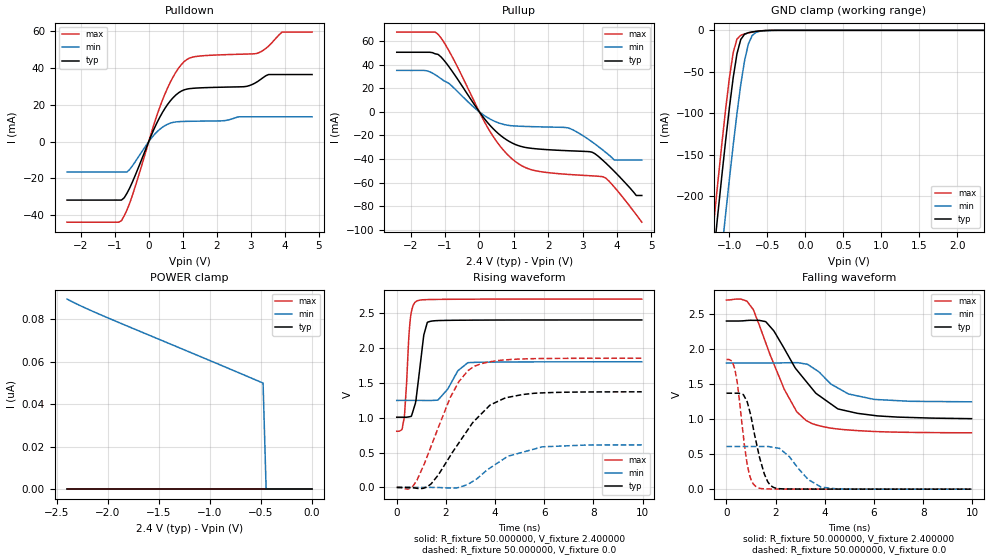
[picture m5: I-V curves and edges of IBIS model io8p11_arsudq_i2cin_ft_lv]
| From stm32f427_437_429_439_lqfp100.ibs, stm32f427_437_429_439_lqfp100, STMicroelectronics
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|   Model io8p11_arsudq_i2cin_ft_lv
[Model]  io8p11_arsudq_i2cin_ft_lv
Model_type I/O
Polarity   Non-Inverting
Enable   Active-Low
Vinl =   0.720000V
Vinh =   1.680000V
Vmeas =  1.200000V
Cref =   30.000000pF
Rref =   100.000000M
Vref =   0.0V
C_comp   2.230300pF   2.174000pF   2.332300pF
[Temperature Range]   25.000000   0.125000k   -40.000000
[Pullup Reference]   2.400000V   1.800000V   2.700000V
[Pulldown Reference]   0.0V   0.0V   0.0V
[POWER Clamp Reference]   2.400000V   1.800000V   2.700000V
[GND Clamp Reference]   0.0V   0.0V   0.0V
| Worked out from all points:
|   slope of the pulldown table from 0 to 0.36 V, typ, clamps not added: 25 ohm
|   slope of the pullup table from 0 to 0.36 V, typ, clamps not added: 27.7 ohm
|   GND clamp passes 1 mA (typ) near -0.62 V on its own axis
|   rising waveform, R_fixture 50.000000, V_fixture 2.400000: 20-80 % time 284ps typ, 604ps min, 184ps max; typ from 1.01 V to 2.4 V
|   rising waveform, R_fixture 50.000000, V_fixture 0.0: 20-80 % time 1.7ns typ, 1.69ns min, 1.31ns max; typ from 0 V to 1.37 V
|   falling waveform, R_fixture 50.000000, V_fixture 2.400000: 20-80 % time 1.81ns typ, 1.28ns min, 1.38ns max; typ from 2.4 V to 1.01 V
|   falling waveform, R_fixture 50.000000, V_fixture 0.0: 20-80 % time 535ps typ, 924ps min, 384ps max; typ from 1.37 V to 0 V
[Pulldown]
|Voltage   I(typ)   I(min)   I(max)
-2.4V     -31.73mA   -16.51mA   -43.74mA
-800mV    -31.73mA   -16.51mA   -42.87mA
-480mV    -21.98mA   -13.17mA   -29.21mA
80mV      3.63mA     1.966mA    5.014mA
480mV     18.16mA    8.738mA    26.02mA
800mV     25.38mA    10.72mA    37.77mA
1.12V     28.53mA    11.02mA    44.6mA
2.8V      29.84mA    13.49mA    47.53mA
3.2V      32.65mA    13.49mA    48.05mA
3.52V     36.43mA    13.49mA    51.84mA
3.92V     36.43mA    13.49mA    59.49mA
4.8V      36.43mA    13.49mA    59.49mA
[Pullup]
|Voltage   I(typ)   I(min)   I(max)
-2.4V     50.45mA    35.08mA    67.53mA
-1.52V    50.45mA    34.74mA    67.53mA
-1.2V     48.64mA    29.87mA    65.68mA
320mV     -11.75mA   -6.207mA   -17.08mA
1.04V     -27.54mA   -11.97mA   -41.91mA
1.6V      -31.14mA   -12.58mA   -49.63mA
2.56V     -32.88mA   -13.48mA   -52.9mA
3.28V     -34.19mA   -25.52mA   -54.18mA
3.6V      -41.31mA   -32.62mA   -54.97mA
3.92V     -50.32mA   -40.8mA    -63.62mA
4.56V     -70.8mA    -40.8mA    -87.08mA
4.72V     -70.8mA    -40.8mA    -93.4mA
[GND_clamp]
|Voltage   I(typ)   I(min)   I(max)
-2.4V     -1.424A    -1.508A    -1.393A
-1.25V    -311.2mA   -401.9mA   -273.3mA
-1.2V     -265.4mA   -356.1mA   -227.2mA
-1.15V    -220.4mA   -310.8mA   -181.9mA
-1.1V     -176.3mA   -266.2mA   -137.9mA
-1.05V    -133.8mA   -222.5mA   -95.87mA
-950mV    -57.3mA    -138.9mA   -26.98mA
-900mV    -28.27mA   -100.4mA   -10.59mA
-850mV    -11.01mA   -65.54mA   -5.958mA
-750mV    -2.834mA   -16.5mA    -3.178mA
-600mV    -750uA     -1.164mA   -738.3uA
2.35V     0A         0A         0A
[POWER_clamp]
|Voltage   I(typ)   I(min)   I(max)
-2.4V     0A         89.62nA    0A
-2.04V    0A         81.57nA    0A
-480mV    0A         50.01nA    0A
-450mV    0A         0A         0A
0V        0A         0A         0A
[Ramp]
| variable   typ   min   max
dV/dt_r  0.82164/1.69610n   0.36402/1.67595n   1.11102/1.31248n
dV/dt_f  0.83178/1.79968n   0.33270/1.30348n   1.13555/1.37499n
R_load = 50.000000
[Rising Waveform]
R_fixture= 50.000000
V_fixture= 2.400000
V_fixture_min= 1.800000
V_fixture_max= 2.700000
|time   V(typ)   V(min)   V(max)
0s        1.006V     1.247V     804.6mV
220.2ps   1.006V     1.247V     837.7mV
300.3ps   1.006V     1.247V     993.4mV
560.6ps   1.015V     1.247V     2.44V
820.8ps   1.362V     1.247V     2.672V
1.101ns   2.185V     1.247V     2.69V
1.261ns   2.369V     1.246V     2.692V
1.682ns   2.391V     1.253V     2.695V
2.903ns   2.397V     1.788V     2.697V
9.97ns    2.4V       1.8V       2.699V
[Rising Waveform]
R_fixture= 50.000000
V_fixture= 0.0
V_fixture_min= 0.0
V_fixture_max= 0.0
|time   V(typ)   V(min)   V(max)
0s        165.6uV    65.51uV    253.7uV
660.7ps   -5.552mV   52.8uV     19.39mV
1.401ns   51.51mV    131.3uV    592.6mV
2.182ns   454.7mV    -7.206mV   1.292V
2.523ns   635.4mV    88.39uV    1.514V
3.123ns   940.4mV    93.01mV    1.729V
3.804ns   1.182V     280.5mV    1.801V
4.424ns   1.284V     424.3mV    1.828V
5.906ns   1.354V     580.2mV    1.847V
9.97ns    1.37V      609mV      1.851V
[Falling Waveform]
R_fixture= 50.000000
V_fixture= 2.400000
V_fixture_min= 1.800000
V_fixture_max= 2.700000
|time   V(typ)   V(min)   V(max)
0s        2.4V       1.8V       2.699V
820.8ps   2.408V     1.8V       2.685V
1.081ns   2.41V      1.8V       2.569V
1.602ns   2.39V      1.8V       2.086V
2.362ns   2V         1.803V     1.419V
2.863ns   1.701V     1.805V     1.104V
3.243ns   1.538V     1.786V     980mV
4.545ns   1.144V     1.442V     858.4mV
6.026ns   1.051V     1.281V     822.9mV
9.97ns    1.006V     1.247V     804.6mV
[Falling Waveform]
R_fixture= 50.000000
V_fixture= 0.0
V_fixture_min= 0.0
V_fixture_max= 0.0
|time   V(typ)   V(min)   V(max)
0s        1.37V      609mV      1.851V
340.3ps   1.37V      609mV      1.716V
440.4ps   1.37V      609mV      1.521V
700.7ps   1.342V     608.9mV    720.6mV
940.9ps   1.12V      608.7mV    199mV
1.261ns   588.9mV    608.7mV    25.75mV
1.682ns   104.9mV    609.6mV    3.118mV
2.042ns   12.22mV    589.2mV    2.071mV
3.844ns   1.143mV    30.16mV    1.067mV
9.97ns    165.6uV    65.51uV    253.7uV
